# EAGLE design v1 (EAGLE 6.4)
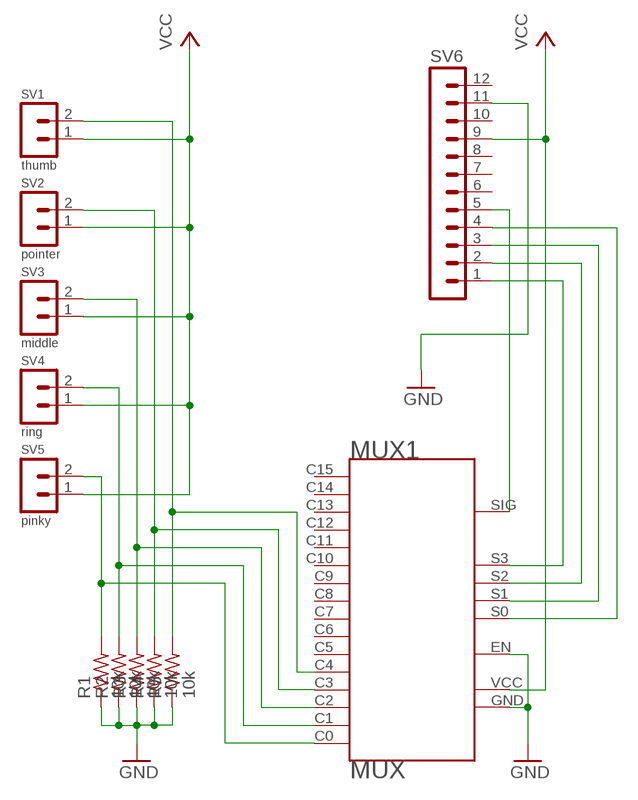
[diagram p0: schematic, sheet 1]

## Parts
MUX1  MUX  [MUX]
R1  10k  R-US_0204/7  [0204/7]
R2  10k  R-US_0204/7  [0204/7]
R3  10k  R-US_0204/7  [0204/7]
R4  10k  R-US_0204/7  [0204/7]
R5  10k  R-US_0204/7  [0204/7]
SV1  thumb  MA02-1  [MA02-1]
SV2  pointer  MA02-1  [MA02-1]
SV3  middle  MA02-1  [MA02-1]
SV4  ring  MA02-1  [MA02-1]
SV5  pinky  MA02-1  [MA02-1]
SV6  MA12-1  [MA12-1]

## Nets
GND: MUX1.EN MUX1.GND R1.1 R2.1 R3.1 R4.1 R5.1 SV6.11
N$2: MUX1.C0 R1.2 SV5.2
N$3: MUX1.C1 R2.2 SV4.2
N$4: MUX1.C2 R3.2 SV3.2
N$5: MUX1.C3 R4.2 SV2.2
N$6: MUX1.C4 R5.2 SV1.2
N$7: MUX1.S2 SV6.2
N$8: MUX1.SIG SV6.5
N$9: MUX1.S3 SV6.1
N$10: MUX1.S1 SV6.3
N$11: MUX1.S0 SV6.4
VCC: MUX1.VCC SV1.1 SV2.1 SV3.1 SV4.1 SV5.1 SV6.9
Unconnected: MUX1.C5 MUX1.C6 MUX1.C7 MUX1.C8 MUX1.C9 MUX1.C10 MUX1.C11 MUX1.C12 MUX1.C13 MUX1.C14 MUX1.C15 SV6.6 SV6.7 SV6.8 SV6.10 SV6.12

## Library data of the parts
MUX1 = Tallent:MUX
R1-R5 = rcl:R-US_: RESISTOR, American symbol
SV1-SV5 = con-lstb:MA02-1: PIN HEADER
SV6 = con-lstb:MA12-1: PIN HEADER; OC_FARNELL: unknown; OC_NEWARK: unknown

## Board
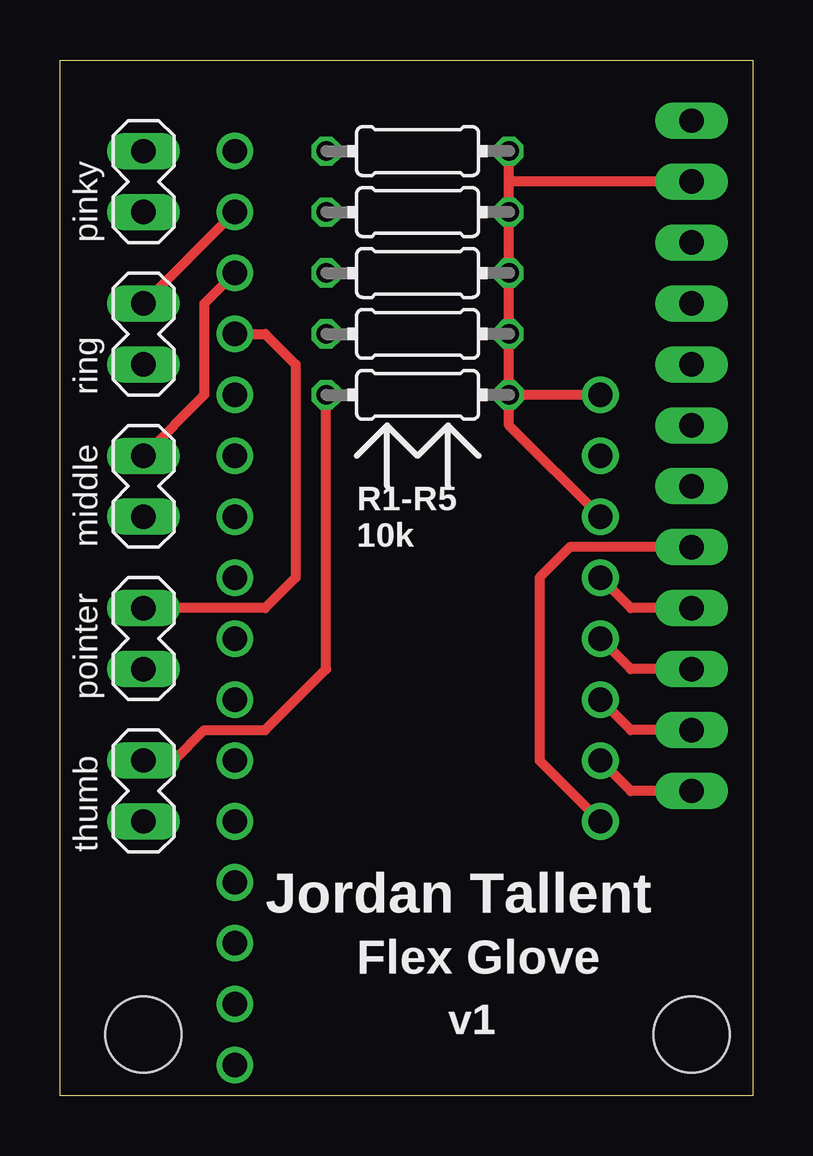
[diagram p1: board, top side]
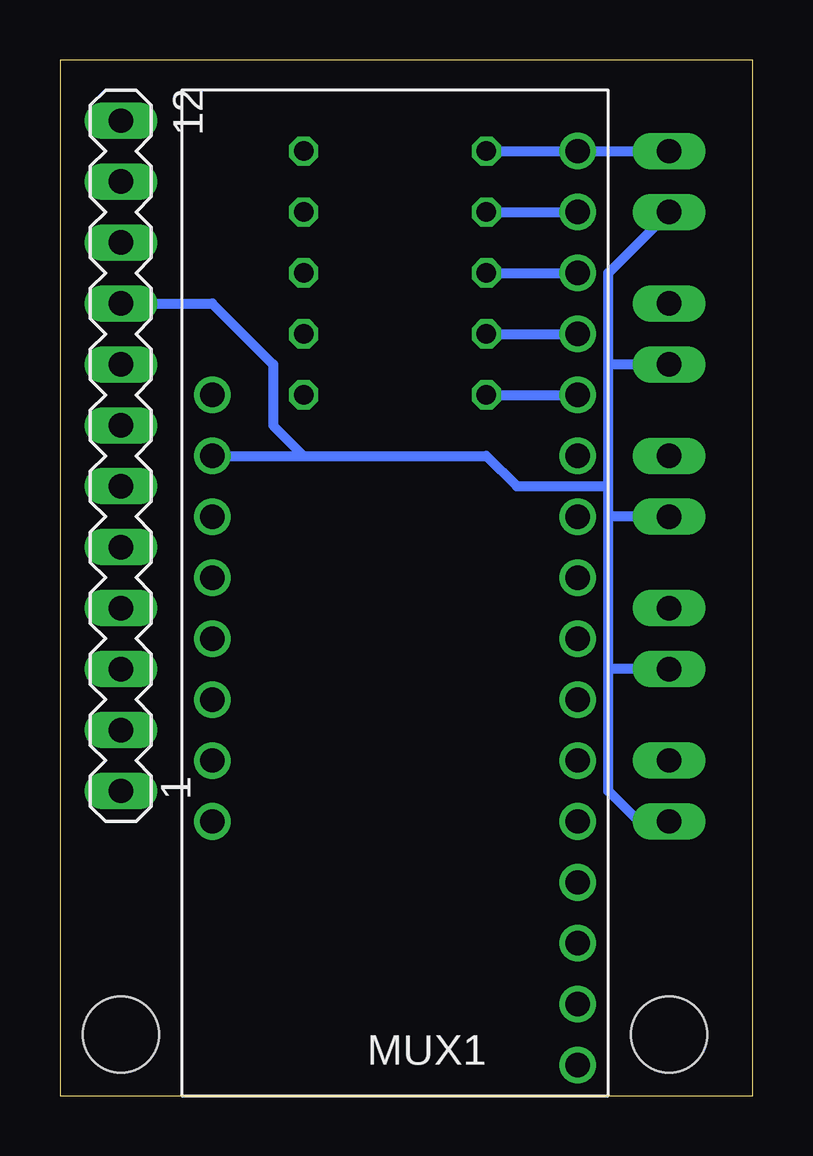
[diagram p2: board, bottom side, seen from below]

Size 28.88 x 43.17 mm. Coordinates in mm from the lower left corner, seen from the top.
Outline: 28.88,0 0,0 0,43.17 28.88,43.17 28.88,0
Copper layers (1*16): Top 0.0356mm / dielectric 1.5011mm / Bottom 0.0356mm
Design rules "OSHpark": minimum track width 6mil, minimum drill 13mil, track to track 6mil, track to pad 6mil, pad to pad 6mil, via to via 6mil, smd to smd 6mil, copper to edge 15mil, drill to drill 6mil, minimum pad ring 7mil, minimum via ring 7mil, stop-mask expansion 4mil, vias tented up to drill 0mil, thermal gap 10mil
Holes 3.17 mm at 26.34,2.54 3.48,2.54

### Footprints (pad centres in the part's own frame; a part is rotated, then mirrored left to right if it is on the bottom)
MUX = drill 1.016: C0 0,-17.78; C1 0,-15.24; C2 0,-12.7; C3 0,-10.16; C4 0,-7.62; C5 0,-5.08; C6 0,-2.54; C7 0,0; C8 0,2.54; C9 0,5.08; C10 0,7.62; C11 0,10.16; C12 0,12.7; C13 0,15.24; C14 0,17.78; C15 0,20.32; EN 15.24,-2.54; GND 15.24,-7.62; S0 15.24,0; S1 15.24,2.54; S2 15.24,5.08; S3 15.24,7.62; SIG 15.24,10.16; VCC 15.24,-5.08
0204/7 = drill 0.813 octagon: 1 -3.81,0; 2 3.81,0
MA02-1 = drill 1.016 long: 1 -1.27,0; 2 1.27,0
MA12-1 = drill 1.016 long: 1 -13.97,0; 2 -11.43,0; 3 -8.89,0; 4 -6.35,0; 5 -3.81,0; 6 -1.27,0; 7 1.27,0; 8 3.81,0; 9 6.35,0; 10 8.89,0; 11 11.43,0; 12 13.97,0

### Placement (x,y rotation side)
MUX1  7.29,21.59 180 bottom
R1  14.91,39.37 180 top
R2  14.91,36.83 180 top
R3  14.91,34.29 180 top
R4  14.91,31.75 180 top
R5  14.91,29.21 180 top
SV1  3.48,12.7 90 top
SV2  3.48,19.05 90 top
SV3  3.48,25.4 90 top
SV4  3.48,31.75 90 top
SV5  3.48,38.1 90 top
SV6  26.34,26.67 90 bottom

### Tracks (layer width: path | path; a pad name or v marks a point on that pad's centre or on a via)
GND
  Top 0.406: MUX1.GND R5.1 | R5.1 R4.1 R3.1 R2.1 18.72,38.1 | SV6.11 18.72,38.1 | 18.72,38.1 R1.1 | MUX1.EN 18.72,27.94 R5.1
N$2
  Bottom 0.406: R1.2 MUX1.C0 SV5.2
N$3
  Top 0.406: SV4.2 MUX1.C1
  Bottom 0.406: R2.2 MUX1.C1
N$4
  Top 0.406: MUX1.C2 6.02,33.02 6.02,29.21 SV3.2
  Bottom 0.406: R3.2 MUX1.C2
N$5
  Top 0.406: MUX1.C3 8.56,31.75 9.83,30.48 9.83,21.59 8.56,20.32 SV2.2
  Bottom 0.406: R4.2 MUX1.C3
N$6
  Top 0.406: SV1.2 4.75,13.97 6.02,15.24 8.56,15.24 11.1,17.78 R5.2
  Bottom 0.406: R5.2 MUX1.C4
N$7
  Top 0.406: SV6.2 23.8,15.24 MUX1.S2
N$8
  Top 0.406: MUX1.SIG 19.99,13.97 19.99,21.59 21.26,22.86 SV6.5
N$9
  Top 0.406: SV6.1 23.8,12.7 MUX1.S3
N$10
  Top 0.406: SV6.3 23.8,17.78 MUX1.S1
N$11
  Top 0.406: SV6.4 23.8,20.32 MUX1.S0
VCC
  Bottom 0.406: MUX1.VCC 18.72,26.67 | 18.72,26.67 11.1,26.67 9.83,25.4 6.02,25.4 | SV1.1 4.75,11.43 6.02,12.7 6.02,17.78 | 6.02,17.78 6.02,24.13 | 6.02,24.13 6.02,25.4 | 6.02,25.4 6.02,30.48 | 6.02,30.48 6.02,34.29 SV5.1 | SV4.1 6.02,30.48 | SV2.1 6.02,17.78 | SV3.1 6.02,24.13 | SV6.9 22.53,33.02 19.99,30.48 19.99,27.94 18.72,26.67

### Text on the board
tNames: R1-R5 / 10k | Jordan Tallent | Flex Glove | v1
